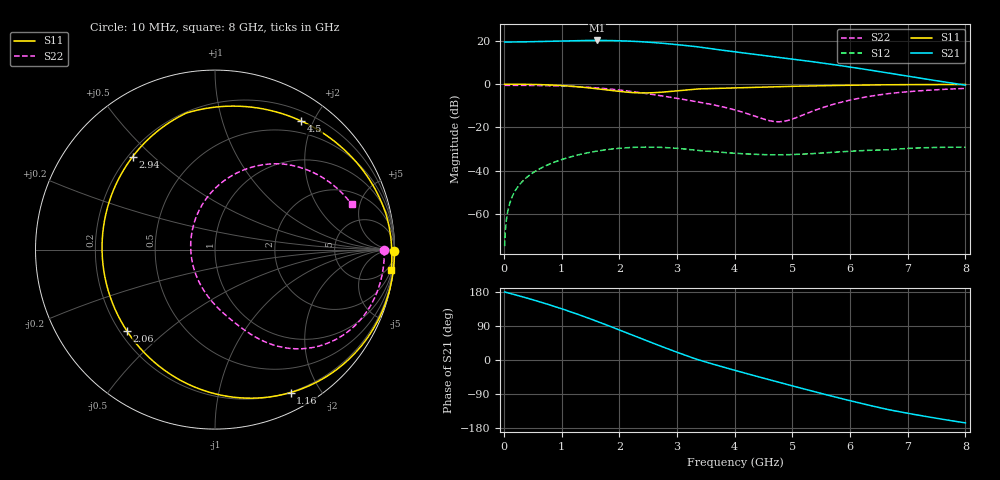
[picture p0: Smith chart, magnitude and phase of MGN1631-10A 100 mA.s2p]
! Port[1] = GATE
! Port[2] = DRAIN
! [Type]  S-parameter s2p file touchstone ver. 1.0
! [Object]  MGN1631-10A
! [Bias]  100 mA
! [Version]  1.0
! [Date]  Thu May 19 10:09:26 2026
! [Source]  This file was created in JSC "ICC Milandr".
! [Disclaimer] Property of JSC "ICC Milandr". Unauthorized reproduction and/or distribution is strictly prohibited.
!  The file and the data are provided "AS IS" and with all faults and disclaim all warranties, express and implied, including
!  without limitation any implied warranties of merchantability, fitness for a particular purpose.
!  JSC "ICC Milandr" assumes no liability for:
!  1) the accuracy of the data provided;
!  2) the proper functioning of this data;
!  3) infringement of patents, copyrights or intellectual property rights resulting from the use of this data.
!  JSC "ICC Milandr" reserves the right to make changes to the products and the data without prior notice.
!  Please, be aware that your receipt and use of the file provided shall serve as acceptance of these terms and conditions.
!  If you do not accept these terms, you should return or destroy this file and any other accompanying information immediately.
# Hz S MA R 12.5
! freq  S11mag  S11ang  S21mag  S21ang  S12mag  S12ang  S22mag  S22ang
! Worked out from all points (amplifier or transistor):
!   800 points, 10 MHz to 8 GHz, reference 12.5 ohm
!   highest |S21| = 20.3 dB at 1.61 GHz (marker M1)
!   |S21| within 3 dB of that: start of sweep to 3.369 GHz
!   unconditionally stable (mu >= 1): 3.903 GHz to 5.076 GHz
!   at 1.34 GHz: K = 0.36, MSG = 26.3 dB, |S12| = -32.4 dB
!   at 4.01 GHz: K = 1.03, MAG = 22.5 dB, |S12| = -32.0 dB
!   at 8 GHz: K = 0.34, MSG = 14.4 dB, |S12| = -29.2 dB
!   S11 on the Smith chart (normalised r, x): 10 MHz: open; 1.16 GHz: 0.19, -1.64; 2.06 GHz: 0.23, -0.37; 2.94 GHz: 0.22, +0.43; 4.5 GHz: 0.33, +1.83; 8 GHz: 2, -17
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1e7  1 -0.4  9.536 179.5  0.0001767 85.3  0.9436 -0.2
8e7  1 -3.8  9.521 176.8  0.001401 86.8  0.9439 -1.7
1.8e8  0.9998 -8.6  9.541 172.7  0.003157 83.7  0.9438 -4.0
6.4e8  0.9789 -31.7  9.786 152.6  0.01139 67.4  0.9339 -14.4
9e8  0.9482 -46.1  9.985 140.1  0.01613 57.2  0.9187 -20.6
1.16e9  0.9009 -62.1  10.17 126.9  0.02083 46.2  0.8938 -27.1
1.35e9  0.8561 -75.2  10.28 116.7  0.02411 37.7  0.8685 -32.0
1.61e9  0.7849 -95.3  10.34 102.1  0.02819 25.4  0.8234 -38.8
1.84e9  0.7202 -115.6  10.29 88.8  0.03118 14.2  0.7738 -44.7
2.06e9  0.6676 -137.5  10.12 75.7  0.0333 3.2  0.7194 -50.2
2.39e9  0.6295 -173.3  9.649 55.9  0.03487 -13.2  0.6304 -57.9
2.68e9  0.6466 155.9  9.054 38.7  0.0346 -27.3  0.5517 -64.0
2.94e9  0.6916 131.6  8.43 23.8  0.03318 -39.3  0.4853 -69.2
3.19e9  0.7453 112.0  7.796 10.0  0.03098 -50.1  0.4265 -74.4
3.43e9  0.7836 97.0  7.132 -2.2  0.02871 -58.3  0.3748 -80.1
3.71e9  0.8044 83.6  6.339 -14.7  0.02684 -63.3  0.3164 -88.6
4.01e9  0.8272 71.7  5.618 -27.6  0.02513 -66.0  0.2524 -101.2
4.5e9  0.8626 56.2  4.649 -47.9  0.02338 -64.8  0.1561 -139.7
5.34e9  0.9149 35.9  3.343 -81.9  0.02464 -55.4  0.2345 112.4
5.98e9  0.9471 23.4  2.529 -106.6  0.02792 -51.9  0.423 77.1
6.67e9  0.9733 11.6  1.813 -131.1  0.03022 -53.8  0.6073 51.8
8e9  0.9883 -6.8  0.9532 -165.9  0.03482 -77.9  0.8016 18.4
